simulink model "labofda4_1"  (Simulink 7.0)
settings: Solver=ode45  SolverMode=SingleTasking  StartTime=0.0  StopTime=30  RelTol=1e-3  AbsTol=1e-6
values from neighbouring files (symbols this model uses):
  A = zeros(5,5)    [labofda4.m]
  b = [0 -32.7 -2.08 0 0]'    [labofda4.m]
  c = [0 0 0 0 1]    [labofda4.m]

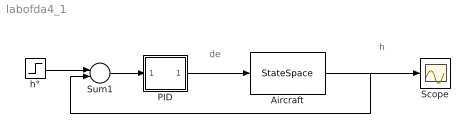
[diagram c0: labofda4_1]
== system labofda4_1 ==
  note: h
  note: de
  Aircraft : StateSpace  A=A  B=b  C=c  D=0  X0=[0 0 0 0 0]
  PID : Subsystem  mask(PID(2) Controller){}
      mask help: Enter Proportional(P), Integral(I), and Derivative(D) and divisor (N) terms. P+I/s+Ds/(1/Ns+1)
      mask init:
      | P=@1; I=@2; D=@3; N=@4;
  Scope : Scope
  Sum1 : Sum  Inputs=+-
  h° : Step  Time=0
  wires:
  Sum1/1 -> PID/1(In_1)
  h°/1 -> Sum1/1
  PID/1(Out_1) -> Aircraft/1
  Aircraft/1 -> Sum1/2, Scope/1

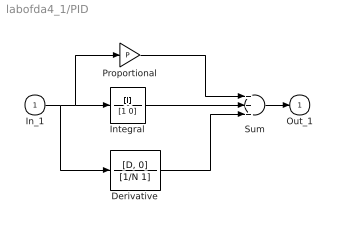
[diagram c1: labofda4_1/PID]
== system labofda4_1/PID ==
  In_1 : Inport
  Derivative : TransferFcn  Numerator=[D, 0]  Denominator=[1/N 1]
  Integral : TransferFcn  Numerator=[I]  Denominator=[1 0]
  Proportional : Gain  Gain=P
  Sum : Sum  Inputs=+++
  Out_1 : Outport  InitialOutput=0
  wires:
  Proportional/1 -> Sum/1
  Integral/1 -> Sum/2
  Derivative/1 -> Sum/3
  In_1/1 -> Integral/1, Proportional/1, Derivative/1
  Sum/1 -> Out_1/1
